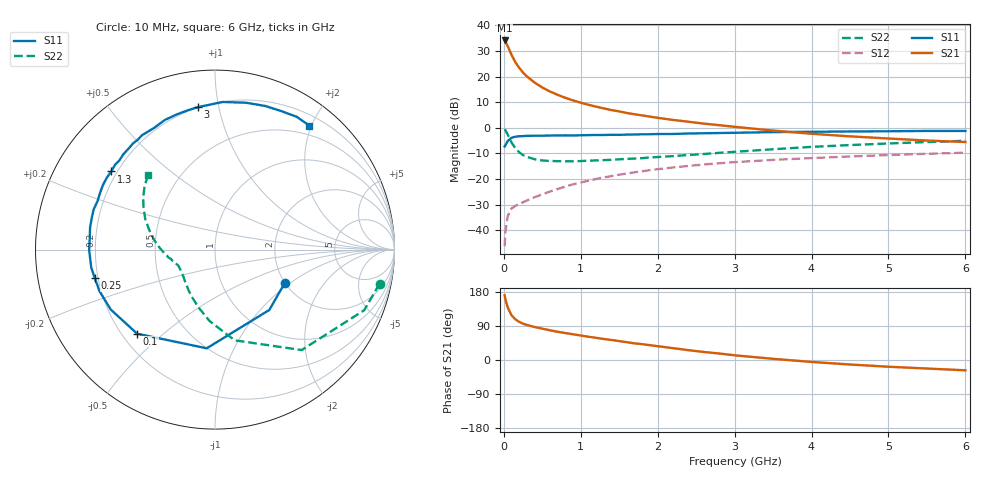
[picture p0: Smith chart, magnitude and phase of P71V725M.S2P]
! SIEMENS Small Signal Semiconductors
! BFP196
! Si NPN RF Bipolar Junction Transistor in SOT143
! VCE = 1.75 V  IC = 25 mA
! Common Emitter S-Parameters:  May  1996
# GHz  S  MA  R  50
!  f  S11  S21  S12  S22
! GHz  MAG  ANG  MAG  ANG  MAG  ANG  MAG  ANG
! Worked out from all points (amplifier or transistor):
!   36 points, 10 MHz to 6 GHz, reference 50 ohm
!   highest |S21| = 34.1 dB at 10 MHz (marker M1)
!   |S21| within 3 dB of that: start of sweep to 61.88 MHz
!   unconditionally stable (mu >= 1): 577.6 MHz to 4.208 GHz
!   at 250 MHz: K = 0.69, MSG = 25.3 dB, |S12| = -29.0 dB
!   at 1.4 GHz: K = 1.11, MAG = 10.9 dB, |S12| = -18.8 dB
!   at 6 GHz: K = 0.98, MSG = 2.1 dB, |S12| = -9.7 dB
!   S11 on the Smith chart (normalised r, x): 10 MHz: 1.99, -0.91; 100 MHz: 0.26, -0.41; 250 MHz: 0.19, -0.11; 1.3 GHz: 0.18, +0.33; 3 GHz: 0.20, +0.87; 6 GHz: 0.35, +1.96
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0.01  0.4307 -25.8  50.63 170.8  0.0049 82.1  0.9367 -11.7
0.02  0.4524 -48.0  48.02 160.7  0.0093 76.1  0.8973 -22.1
0.05  0.5519 -94.8  39.39 138.9  0.0189 57.4  0.7393 -49.2
0.1  0.6385 -132.8  26.46 118.1  0.0266 44.8  0.5171 -77.8
0.15  0.67 -150.1  19.03 107.2  0.03 41.9  0.3984 -94.5
0.2  0.6837 -160.1  14.79 100.5  0.0325 41.8  0.3326 -106.5
0.25  0.6887 -166.8  11.92 95.8  0.0353 43.6  0.2932 -116.0
0.3  0.6967 -171.8  10.04 92.4  0.0382 45.4  0.2715 -122.7
0.4  0.7012 -179.8  7.627 87.1  0.0443 49.0  0.2436 -133.2
0.5  0.7006 175.1  6.107 82.6  0.0501 51.8  0.2305 -140.4
0.6  0.7069 169.9  5.101 78.4  0.0571 53.5  0.2253 -145.5
0.7  0.7092 165.2  4.392 74.4  0.064 54.7  0.2231 -149.4
0.9  0.708 157.4  3.423 67.9  0.0789 55.3  0.2222 -155.1
1.1  0.7204 150.2  2.816 61.4  0.0926 55.2  0.228 -158.8
1.3  0.7235 143.0  2.389 55.4  0.1077 53.7  0.234 -162.3
1.7  0.7406 130.5  1.834 43.9  0.1354 50.2  0.2511 -168.2
2.2  0.758 116.6  1.424 31.2  0.1682 44.0  0.2802 -175.1
3  0.7993 96.9  1.044 12.4  0.2137 33.4  0.3398 171.7
3.5  0.8236 87.0  0.883 3.1  0.2364 26.8  0.3815 163.6
4.5  0.8478 70.7  0.681 -11.9  0.2761 15.3  0.4605 149.8
5.5  0.8689 58.4  0.564 -22.5  0.3109 4.5  0.5278 138.0
6  0.8679 52.8  0.528 -27.2  0.3272 -1.3  0.5574 132.2
